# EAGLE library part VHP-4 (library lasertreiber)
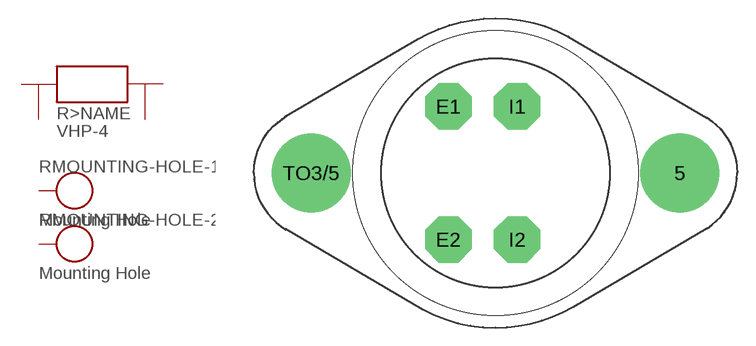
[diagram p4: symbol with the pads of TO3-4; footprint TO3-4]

Designator prefix R; gates >NAME=R-4WIRE MOUNTING-HOLE-1=MOUNTING-HOLES MOUNTING-HOLE-2=MOUNTING-HOLES

## VHP-4  [TO3-4]
5  MOUNTING-HOLE-1:1
E1  >NAME:E1
E2  >NAME:E2
I1  >NAME:I1
I2  >NAME:I2
TO3/5  MOUNTING-HOLE-2:1

## Footprint TO3-4 (pad centres in mm)
VOLTAGE REGULATOR
drill 4.115 pad 6.477: 5 15.113,0; TO3/5 -15.113,0
drill 1.194 pad 3.81 octagon: E1 -3.861,5.461; E2 -3.861,-5.461; I1 1.778,5.461; I2 1.778,-5.461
